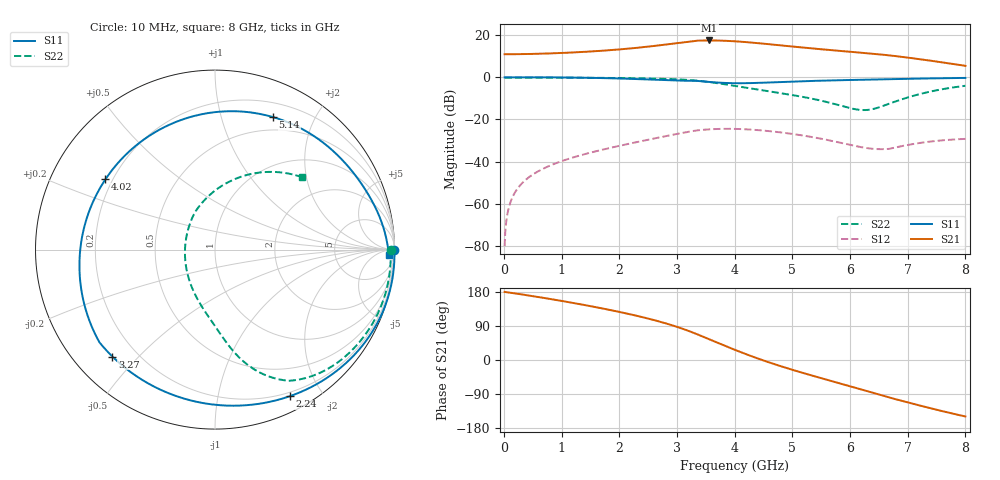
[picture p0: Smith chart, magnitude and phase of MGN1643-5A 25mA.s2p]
! Port[1] = GATE
! Port[2] = DRAIN
! [Type]  S-parameter s2p file touchstone ver. 1.0
! [Object]  MGN1643-5A
! [Bias]  25 mA
! [Version]  1.0
! [Date]  Thu May 19 10:56:59 2026
! [Source]  This file was created in JSC "ICC Milandr".
! [Disclaimer] Property of JSC "ICC Milandr". Unauthorized reproduction and/or distribution is strictly prohibited.
!  The file and the data are provided "AS IS" and with all faults and disclaim all warranties, express and implied, including
!  without limitation any implied warranties of merchantability, fitness for a particular purpose.
!  JSC "ICC Milandr" assumes no liability for:
!  1) the accuracy of the data provided;
!  2) the proper functioning of this data;
!  3) infringement of patents, copyrights or intellectual property rights resulting from the use of this data.
!  JSC "ICC Milandr" reserves the right to make changes to the products and the data without prior notice.
!  Please, be aware that your receipt and use of the file provided shall serve as acceptance of these terms and conditions.
!  If you do not accept these terms, you should return or destroy this file and any other accompanying information immediately.
# Hz S MA R 12.5
! freq  S11mag  S11ang  S21mag  S21ang  S12mag  S12ang  S22mag  S22ang
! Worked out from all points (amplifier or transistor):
!   800 points, 10 MHz to 8 GHz, reference 12.5 ohm
!   highest |S21| = 17.5 dB at 3.56 GHz (marker M1)
!   |S21| within 3 dB of that: 2.475 GHz to 5.044 GHz (2.569 GHz wide, 68.3 % of centre)
!   unconditionally stable (mu >= 1): 5.765 GHz to 6.941 GHz
!   at 1.34 GHz: K = 0.20, MSG = 24.5 dB, |S12| = -36.9 dB
!   at 4.01 GHz: K = 0.53, MSG = 20.8 dB, |S12| = -24.5 dB
!   at 8 GHz: K = 0.48, MSG = 17.3 dB, |S12| = -29.2 dB
!   S11 on the Smith chart (normalised r, x): 10 MHz: open; 2.24 GHz: 0.16, -1.62; 3.27 GHz: 0.11, -0.42; 4.02 GHz: 0.17, +0.28; 5.14 GHz: 0.35, +1.47; 8 GHz: 32, -32
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1e7  1 -0.2  3.531 179.8  9.834e-05 86.8  0.9784 -0.1
1.1e8  1.001 -2.4  3.534 177.6  0.001073 87.7  0.9792 -1.4
3.1e8  1.002 -6.9  3.559 173.0  0.003039 84.3  0.9806 -4.1
1.35e9  0.9813 -32.4  3.996 146.4  0.01442 63.3  0.9775 -18.6
2.24e9  0.917 -63.0  4.925 118.8  0.02787 40.5  0.9541 -33.3
2.68e9  0.8714 -85.8  5.72 102.1  0.03715 25.9  0.9293 -42.5
2.98e9  0.8418 -107.0  6.435 88.5  0.04486 13.6  0.9002 -50.0
3.27e9  0.8257 -133.8  7.224 72.7  0.05302 -1.1  0.8536 -58.4
3.38e9  0.8161 -145.2  7.444 66.0  0.05568 -7.3  0.8271 -61.8
3.56e9  0.777 -163.7  7.507 54.6  0.05827 -17.5  0.7724 -66.6
3.79e9  0.7407 171.6  7.413 40.0  0.05993 -30.2  0.6968 -72.2
4.01e9  0.7255 148.4  7.163 26.4  0.05974 -41.6  0.6248 -76.8
4.02e9  0.7253 147.4  7.149 25.8  0.05969 -42.1  0.6216 -77.0
4.28e9  0.7305 122.5  6.715 10.7  0.05749 -54.2  0.5443 -81.6
4.59e9  0.7548 97.9  6.128 -6.0  0.053 -66.2  0.4662 -86.7
4.86e9  0.7806 80.7  5.63 -19.3  0.04811 -74.5  0.4077 -91.8
5.14e9  0.8058 66.4  5.161 -32.2  0.04249 -81.0  0.3513 -98.9
5.34e9  0.8219 57.8  4.861 -41.0  0.03828 -84.1  0.3115 -105.6
5.98e9  0.8637 36.8  4.066 -68.4  0.02527 -82.6  0.1888 -148.3
6.67e9  0.9047 20.8  3.337 -98.6  0.02 -53.1  0.2363 118.2
7.29e9  0.9388 10.0  2.603 -123.3  0.02871 -53.9  0.4269 71.0
8e9  0.9688 -1.8  1.876 -149.0  0.03463 -67.7  0.6301 39.9
